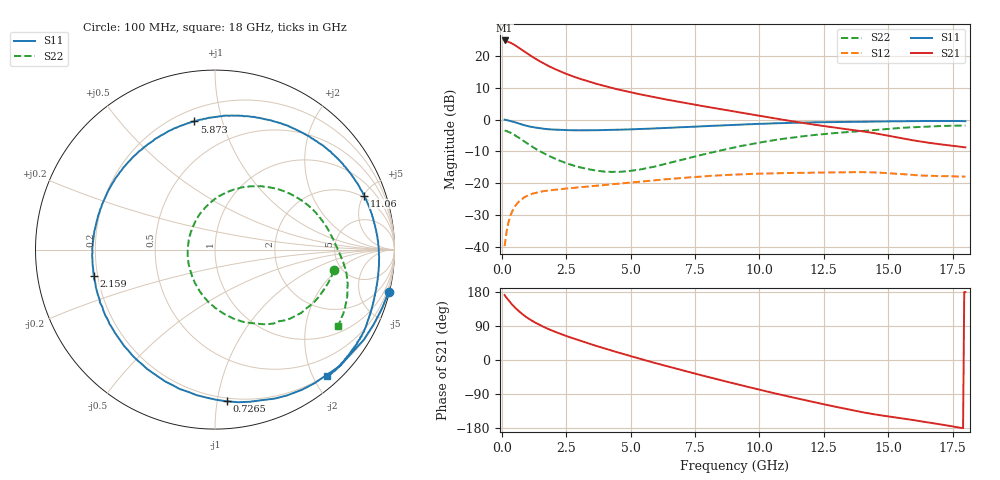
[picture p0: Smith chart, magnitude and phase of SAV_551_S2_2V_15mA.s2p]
! Data provided by Modelithics, Inc.  Tampa, Florida USA, June 2008
!Model SAV-551+
!VAR V_out= 2
!VAR I_out= 15
!VAR V_in= 0.3343
!VAR I_in= 0.8873
!BEGIN ACDATA
# GHZ S MA R 50
! Scattering Parameters
!% F n11x n11y n21x n21y n12x n12y n22x n22y
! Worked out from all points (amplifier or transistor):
!   401 points, 100 MHz to 18 GHz, reference 50 ohm
!   highest |S21| = 24.8 dB at 100 MHz (marker M1)
!   |S21| within 3 dB of that: start of sweep to 780.4 MHz
!   unconditionally stable (mu >= 1): 4.525 GHz to 10.66 GHz
!   at 3.054 GHz: K = 0.78, MSG = 16.9 dB, |S12| = -21.2 dB
!   at 9.05 GHz: K = 1.07, MAG = 8.2 dB, |S12| = -17.2 dB
!   at 18 GHz: K = 0.89, MSG = 4.6 dB, |S12| = -17.9 dB
!   lowest NFmin = 0.08 dB at 500 MHz
!   S11 on the Smith chart (normalised r, x): 100 MHz: 0.15, -8.33; 726.5 MHz: 0.18, -1.06; 2.159 GHz: 0.18, -0.10; 5.873 GHz: 0.27, +0.82; 11.06 GHz: 1.83, +5.04; 18 GHz: 0.17, -2.21
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0.1  0.9959 -13.7  17.29 171.4  0.01043 84.7  0.6709 -9.9
0.14475  0.9867 -19.3  16.75 166.9  0.01397 79.8  0.6662 -12.8
0.23425  0.9694 -31.2  16.5 159.3  0.02325 72.3  0.6443 -21.0
0.32375  0.9519 -42.8  15.99 151.9  0.03121 67.2  0.6232 -28.7
0.41325  0.9279 -53.5  15.3 144.7  0.03798 61.6  0.5957 -36.3
0.5475  0.8945 -68.1  14.16 135.6  0.04599 53.9  0.5528 -45.5
0.7265  0.8477 -85.6  12.66 124.6  0.05558 45.5  0.4953 -57.1
0.995  0.7909 -107.5  10.7 110.8  0.06445 36.5  0.4174 -71.2
1.30825  0.748 -128.0  8.903 98.1  0.07099 28.6  0.3474 -84.8
1.711  0.7127 -149.1  7.219 84.5  0.07658 21.4  0.2839 -99.7
2.1585  0.6913 -167.7  5.919 71.8  0.08046 15.7  0.2347 -114.3
2.56125  0.6821 178.3  5.071 61.7  0.08389 11.3  0.2036 -126.7
3.09825  0.6765 162.0  4.248 49.4  0.08778 7.0  0.1757 -143.4
4.396  0.6895 129.5  3.034 22.1  0.09798 -3.1  0.152 174.2
5.87275  0.7233 99.1  2.252 -6.5  0.1112 -14.5  0.1809 130.7
6.0965  0.7312 95.0  2.165 -10.6  0.1134 -16.5  0.1912 125.1
7.439  0.7726 72.0  1.721 -34.9  0.1253 -28.6  0.2603 96.3
9.05  0.8244 47.6  1.327 -62.5  0.1379 -44.6  0.3672 68.6
11.06375  0.8837 19.9  0.9711 -95.3  0.1453 -66.6  0.5083 39.1
12.04825  0.9017 7.8  0.8417 -110.1  0.1474 -77.5  0.5689 26.7
15.0465  0.9369 -23.5  0.5548 -149.4  0.1445 -107.7  0.7158 -5.4
18  0.9435 -48.5  0.3668 179.1  0.1278 -132.7  0.8058 -31.9
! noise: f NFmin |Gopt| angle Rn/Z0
0.5  0.083  0.3404  26.36  0.086
0.7  0.118  0.3559  36.66  0.077
0.9  0.153  0.3706  46.8  0.068
1  0.171  0.3777  51.81  0.064
1.9  0.329  0.4336  95.22  0.039
2.4  0.417  0.4585  118  0.033
3  0.523  0.4826  144.1  0.034
3.9  0.682  0.5068  -179.3  0.051
5  0.875  0.517  -138.8  0.098
6  1.051  0.5077  -106  0.164
